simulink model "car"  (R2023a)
settings: Solver=ode15s  StartTime=0.0  StopTime=60  RelTol=1e-3  EnableMultiTasking=on
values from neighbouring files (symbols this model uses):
  A_a = 1.5    [modelparam.m]
  b_f = 0.1    [modelparam.m]
  b_t = 0.1    [modelparam.m]
  brake_gain = 1.0e3    (= 1000)    [modelparam.m]
  Bx = Kxk/(Cx*Dx)    (= 12.5)    [modelparam.m]
  c_c = 30    [modelparam.m]
  c_d = 1    [modelparam.m]
  c_p = 15    [modelparam.m]
  c_r = 0.015    [modelparam.m]
  c_w = 0.30    (= 0.3)    [modelparam.m]
  Cx = 1.2    [modelparam.m]
  Dx = muX*Fz    (= 5886)    [modelparam.m]
  Ex = 0.8    [modelparam.m]
  g = 9.81    [modelparam.m]
  gearInertia = [0.13 0.09 0.07 0.05 0.04]    [modelparam.m]
  gearNumber = [1 2 3 4 5]    [modelparam.m]
  gearRatio = [3.4 2.2 1.5 1.1 0.9]    [modelparam.m]
  i_f = 3.4    [modelparam.m]
  IdleControllerI = 0.2    [modelparam.m]
  IdleControllerP = 0.8    [modelparam.m]
  init_d = init_v/r_w/3.6    (= 27.7777777778)    [modelparam.m]
  init_e = init_t*gearRatio(2)    [modelparam.m]
  init_f = init_d    (= 27.7777777778)    [modelparam.m]
  init_t = init_f*i_f    (= 94.4444444444)    [modelparam.m]
  init_T = 0    [modelparam.m]
  J_e = 0.2    [modelparam.m]
  J_f = 0.1    [modelparam.m]
  J_w = 0.6    [modelparam.m]
  k_c = 10e3    (= 10000)    [modelparam.m]
  k_d = 1e3    (= 1000)    [modelparam.m]
  k_p = 0.5e4    (= 5000)    [modelparam.m]
  mass = 1.5e3    (= 1500)    [modelparam.m]
  N_idle = 8.5e2*pi/30    (= 89.0117918517)    [modelparam.m]
  N_max = 7e3*pi/30    (= 733.038285838)    [modelparam.m]
  position = [0 1e6]    [modelparam.m]
  r_w = 0.30    (= 0.3)    [modelparam.m]
  Rho_a = 1.29    [modelparam.m]
  slope = [0 0]    [modelparam.m]
  T_max = 400    [modelparam.m]
  tau_d = 1e-3    (= 0.001)    [modelparam.m]
  tau_e = 0.1    [modelparam.m]
libraries: simulink x4

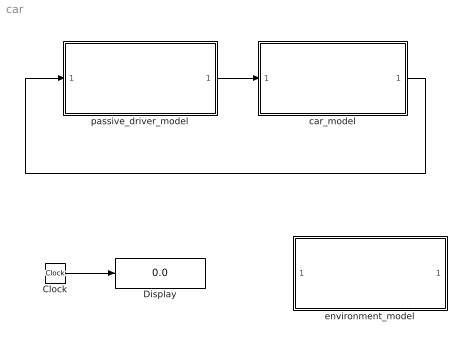
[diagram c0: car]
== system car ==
  Clock : Clock
  Display : Display
  car_model : Subsystem
  environment_model : Subsystem  AncestorBlock=capsim_lib/Environment/environment_model_jofr1  mask{Tamb=0, Pamb=0, pos=position, slope=slope}
      mask prompts: Tamb "Ambient Temperature [K]"; Pamb "Ambient Pressure [Pa]"; pos "positionvector in slope map [m]"; slope "slopevector in slope map [rad]"
      mask help: Environment settings
  passive_driver_model : Subsystem  AncestorBlock=capsim_lib/Driver/driver_model_template
      mask help: Driver model
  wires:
  car_model/1(vehicle fb out) -> passive_driver_model/1(vehicle fb in)
  passive_driver_model/1(driver cmd out) -> car_model/1(driver cmd in)
  Clock/1 -> Display/1

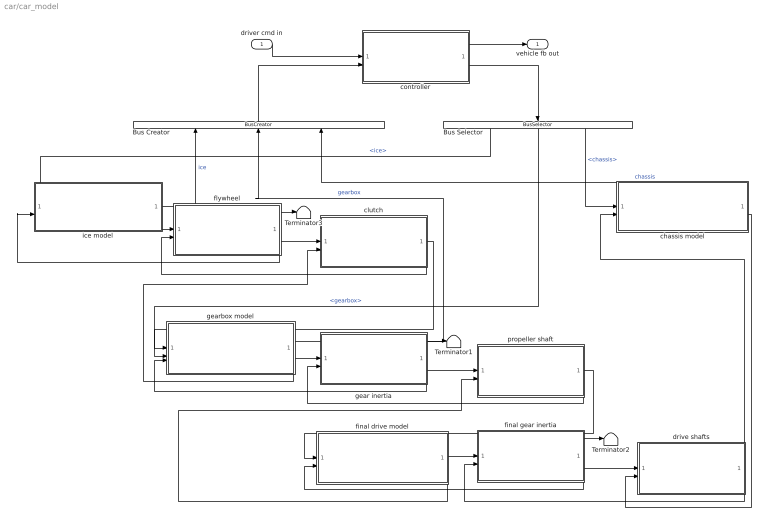
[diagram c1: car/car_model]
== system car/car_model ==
  driver cmd in : Inport
  Bus Creator : BusCreator  Inputs=3
  Bus Selector : BusSelector  OutputSignals=ice,gearbox,chassis
  Terminator1 : Terminator
  Terminator2 : Terminator
  Terminator3 : Terminator
  chassis model : Subsystem  AncestorBlock=capsim_lib/Chassis/chassis_model_template
  clutch : Subsystem  AncestorBlock=capsim_lib/MechConverter/mechconverter_simple1_std  mask{mass=0, inertia=0, k_c=k_c, c_c=c_c}
      mask prompts: mass "Component mass [kg]"; inertia "Inertia [kg*m2]"; k_c "stiffness [Nm/rad]"; c_c "damping [Nms/rad]"
      mask help: Inertia
  controller : Subsystem  AncestorBlock=capsim_lib/Controller/controller_template
  drive shafts : Subsystem  AncestorBlock=capsim_lib/MechConverter/mechconverter_simple1_std  mask{mass=0, inertia=0, k_d=k_d, c_d=c_d}
      mask prompts: mass "Component mass [kg]"; inertia "Inertia [kg*m2]"; k_d "stiffness [Nm/rad]"; c_d "damping [Nms/rad]"
      mask help: Inertia
  final drive model : Subsystem  AncestorBlock=capsim_lib/Gearbox/gearbox_template
  final gear inertia : Subsystem  AncestorBlock=capsim_lib/Inertia/inertia_simple1_std  mask{mass=0, inertia=0, speedinit=init_f, angleinit=0}
      mask prompts: mass "Component mass [kg]"; inertia "Inertia [kg*m2]"; speedinit "Initial speed [rad/s]"; angleinit "Initial angle [rad]"
      mask help: Inertia
  flywheel : Subsystem  AncestorBlock=capsim_lib/Inertia/inertia_simple1_std  mask{mass=0, inertia=0, speedinit=init_e, angleinit=0}
      mask prompts: mass "Component mass [kg]"; inertia "Inertia [kg*m2]"; speedinit "Initial speed [rad/s]"; angleinit "Initial angle [rad]"
      mask help: Inertia
  gear inertia : Subsystem  AncestorBlock=capsim_lib/Inertia/inertia_simple1_std  mask{mass=0, inertia=0, speedinit=init_t, angleinit=0}
      mask prompts: mass "Component mass [kg]"; inertia "Inertia [kg*m2]"; speedinit "Initial speed [rad/s]"; angleinit "Initial angle [rad]"
      mask help: Inertia
  gearbox model : Subsystem  AncestorBlock=capsim_lib/Gearbox/gearbox_template
  ice model : Subsystem
  propeller shaft : Subsystem  AncestorBlock=capsim_lib/MechConverter/mechconverter_simple1_std  mask{mass=0, inertia=0, k_p=k_p, c_p=c_p}
      mask prompts: mass "Component mass [kg]"; inertia "Inertia [kg*m2]"; k_p "stiffness [Nm/rad]"; c_p "damping [Nms/rad]"
      mask help: Inertia
  vehicle fb out : Outport
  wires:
  controller/1(vehicle fb out) -> vehicle fb out/1
  driver cmd in/1 -> controller/1(driver cmd in)
  controller/2(cmd out) -> Bus Selector/1
  Bus Creator/1 -> controller/2(sensor in)
  Bus Selector/1 -> ice model/1(cmd in)  "<ice>"
  Bus Selector/3 -> chassis model/1(cmd in)  "<chassis>"
  chassis model/1(sensor out) -> Bus Creator/3  "chassis"
  ice model/2(mech power out [Nm]) -> flywheel/1(mech in [Nm])
  flywheel/3(mech fb out [rad/s]) -> ice model/2(mech fb in [rad/s])
  flywheel/2(mech out [rad/s]) -> clutch/1(mech in [rad/s])
  clutch/2(mech fb out [Nm]) -> flywheel/2(mech fb in [Nm])
  clutch/1(mech out [Nm]) -> gearbox model/2(mech power in [Nm])
  gearbox model/2(mech power out [Nm]) -> gear inertia/1(mech in [Nm])
  gearbox model/3(mech fb out [rad/s]) -> clutch/2(mech fb in [rad/s])
  gear inertia/3(mech fb out [rad/s]) -> gearbox model/3(mech fb in [rad/s])
  gear inertia/2(mech out [rad/s]) -> propeller shaft/1(mech in [rad/s])
  propeller shaft/2(mech fb out [Nm]) -> gear inertia/2(mech fb in [Nm])
  propeller shaft/1(mech out [Nm]) -> final drive model/1(mech power in [Nm])
  final drive model/2(mech fb out [rad/s]) -> propeller shaft/2(mech fb in [rad/s])
  final drive model/1(mech power out [Nm]) -> final gear inertia/1(mech in [Nm])
  final gear inertia/2(mech out [rad/s]) -> drive shafts/1(mech in [rad/s])
  final gear inertia/3(mech fb out [rad/s]) -> final drive model/2(mech fb in [rad/s])
  drive shafts/1(mech out [Nm]) -> chassis model/2(mech power in [Nm])
  drive shafts/2(mech fb out [Nm]) -> final gear inertia/2(mech fb in [Nm])
  chassis model/2(mech fb out [rad/s]) -> drive shafts/2(mech fb in [rad/s])
  ice model/1(sensor out) -> Bus Creator/1  "ice"
  flywheel/1(sensor out) -> Terminator3/1
  gearbox model/1(sensor out) -> Bus Creator/2  "gearbox"
  gear inertia/1(sensor out) -> Terminator1/1
  final gear inertia/1(sensor out) -> Terminator2/1
  Bus Selector/2 -> gearbox model/1(cmd in)  "<gearbox>"

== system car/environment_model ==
  Compare To Constant : simulink/Logic and Bit Operations/Compare To Constant  relop=<  const=1  OutDataTypeStr=uint8  ZeroCross=off
  Compare To Constant1 : simulink/Logic and Bit Operations/Compare To Constant  relop=<  const=1  OutDataTypeStr=uint8  ZeroCross=off
  Constant2 : Constant  Value=pos(end)
  Integrator : Integrator
  Logical Operator : Logic  Operator=OR  Inputs=3  AllPortsSameDT=off  OutDataTypeStr=boolean
  Relational Operator : RelationalOperator
  Stop Simulation1 : Stop
  To Workspace2 : ToWorkspace  VariableName=environmentout  SampleTime=-1
  slope as function of the distance : Lookup  InputValues=pos  Table=slope  LookUpMeth=Interpolation-Use End Values
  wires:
  [speed] -> Integrator/1, Compare To Constant/1
  Integrator/1 -> slope as function of the distance/1, Relational Operator/1  "distance"
  slope as function of the distance/1 -> [slope], To Workspace2/1
  Constant2/1 -> Relational Operator/2
  Logical Operator/1 -> Stop Simulation1/1
  Relational Operator/1 -> Logical Operator/1
  Compare To Constant/1 -> Logical Operator/2
  [wheelspeed] -> Compare To Constant1/1
  Compare To Constant1/1 -> Logical Operator/3

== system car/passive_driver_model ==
  vehicle fb in : Inport
  Bus Creator : BusCreator  Inputs=1
  Bus Selector : BusSelector  OutputSignals=velocity [m/s]
  From Workspace2 : FromWorkspace  VariableName=[InputT InputU]
  Terminator : Terminator
  driver cmd out : Outport
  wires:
  vehicle fb in/1 -> Bus Selector/1
  Bus Creator/1 -> driver cmd out/1
  Bus Selector/1 -> Terminator/1  "<velocity [m/s]>"
  From Workspace2/1 -> Bus Creator/1  "Torque demand [%]"

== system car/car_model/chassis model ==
  cmd in : Inport
  mech power in [Nm] : Inport  Port=2
  chassis : Subsystem  mask{g=g, mass=mass, J_w=J_w, r_w=r_w, init_d=init_d, c_w=c_w, A_a=A_a, Rho_a=Rho_a, c_r=c_r, Bx=Bx, Cx=Cx, Dx=Dx, Ex=Ex}
      mask prompts: g "gravity constant [m/s^2]"; mass "vehicle mass [kg]"; J_w "wheel inertia [kg m^2]"; r_w "wheel radius [m]"; init_d "initial drive shaft speed [rad/s]"; c_w "air drag coefficient [-]"; A_a "max. vehicle cross section area [m^2]"; Rho_a "Air density [kg/m^3]"; c_r "rolling resistance coefficient [-]"; Bx "Magic Bx"; Cx "Magic Cx"; Dx "Magic Dx"; Ex "Magic Ex"
  local controller : Subsystem  mask{brake_gain=brake_gain}
      mask prompts: brake_gain "brake gain [Nm]"
  sensor out : Outport
  mech fb out [rad/s] : Outport  Port=2
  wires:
  local controller/2(ctrl out) -> chassis/1(ctrl in)
  cmd in/1 -> local controller/1(cmd in)
  local controller/1(sensor out) -> sensor out/1
  chassis/1(sensor out) -> local controller/2(sensor in)
  mech power in [Nm]/1 -> chassis/2(mech power in [Nm])
  chassis/2(mech fb out [rad/s]) -> mech fb out [rad/s]/1

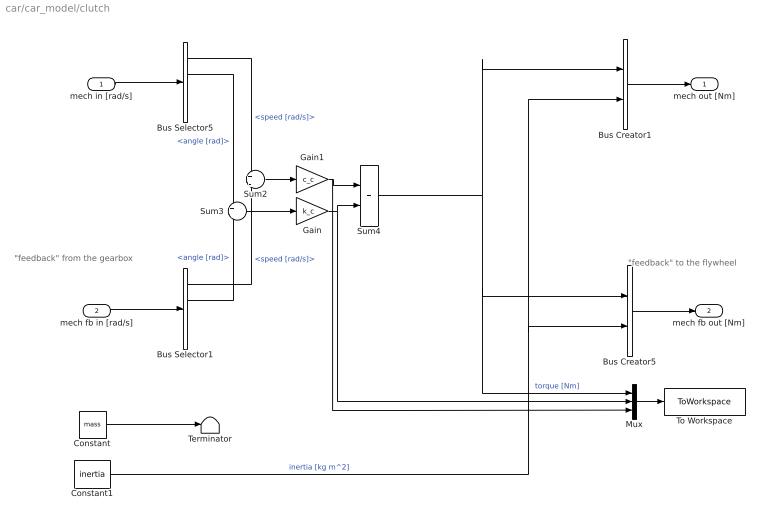
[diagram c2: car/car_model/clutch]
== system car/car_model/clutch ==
  note: "feedback" from the gearbox
  note: "feedback" to the flywheel
  mech in [rad/s] : Inport
  mech fb in [rad/s] : Inport  Port=2
  Bus Creator1 : BusCreator  Inputs=2
  Bus Creator5 : BusCreator  Inputs=2
  Bus Selector1 : BusSelector  OutputSignals=speed [rad/s],angle [rad]
  Bus Selector5 : BusSelector  OutputSignals=speed [rad/s],angle [rad]
  Constant : Constant  Value=mass
  Constant1 : Constant  Value=inertia
  Gain : Gain  Gain=k_c
  Gain1 : Gain  Gain=c_c
  Mux : Mux  Inputs=3
  Sum2 : Sum  Inputs=+|-  SaturateOnIntegerOverflow=on
  Sum3 : Sum  Inputs=+|-  SaturateOnIntegerOverflow=on
  Sum4 : Sum
  Terminator : Terminator
  To Workspace : ToWorkspace  VariableName=clutchout  SampleTime=-1
  mech out [Nm] : Outport
  mech fb out [Nm] : Outport  Port=2
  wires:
  mech in [rad/s]/1 -> Bus Selector5/1
  mech fb in [rad/s]/1 -> Bus Selector1/1
  Mux/1 -> To Workspace/1
  Constant/1 -> Terminator/1
  Bus Creator5/1 -> mech fb out [Nm]/1
  Bus Creator1/1 -> mech out [Nm]/1
  Bus Selector5/1 -> Sum2/1  "<speed [rad/s]>"
  Bus Selector5/2 -> Sum3/1  "<angle [rad]>"
  Bus Selector1/1 -> Sum2/2  "<speed [rad/s]>"
  Bus Selector1/2 -> Sum3/2  "<angle [rad]>"
  Sum2/1 -> Gain1/1
  Sum3/1 -> Gain/1
  Gain1/1 -> Sum4/1, Mux/3
  Gain/1 -> Sum4/2, Mux/2
  Sum4/1 -> Bus Creator1/1, Bus Creator5/1, Mux/1  "torque [Nm]"
  Constant1/1 -> Bus Creator5/2, Bus Creator1/2  "inertia [kg m^2]"

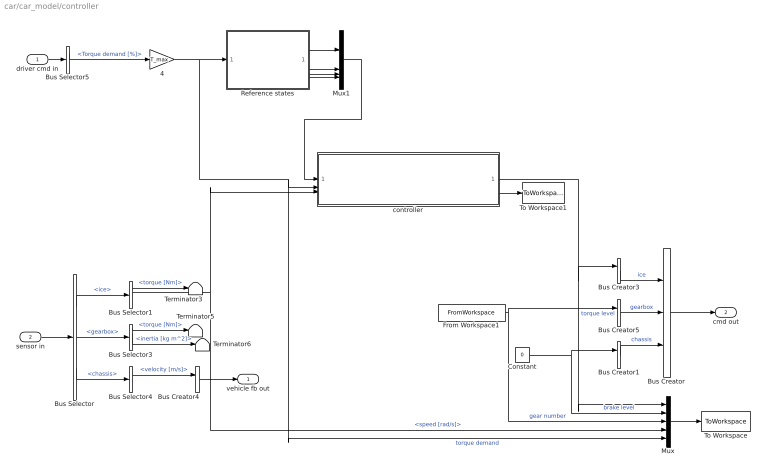
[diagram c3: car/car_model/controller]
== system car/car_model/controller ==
  driver cmd in : Inport
  sensor in : Inport  Port=2
  4 : Gain  Gain=T_max
  Bus Creator : BusCreator  Inputs=3
  Bus Creator{1,3..5} (4 alike) : BusCreator  Inputs=1
  Bus Selector : BusSelector  OutputSignals=ice,gearbox,chassis
  Bus Selector1 : BusSelector  OutputSignals=torque [Nm],speed [rad/s]
  Bus Selector3 : BusSelector  OutputSignals=torque [Nm],inertia [kg m^2]
  Bus Selector4 : BusSelector  OutputSignals=velocity [m/s]
  Bus Selector5 : BusSelector  OutputSignals=Torque demand [%]
  Constant : Constant  Value=0
  From Workspace1 : FromWorkspace  VariableName=[InputT InputG]
  Mux : Mux  Inputs=5
  Mux1 : Mux
  Reference states : Subsystem
  Terminator3 : Terminator
  Terminator5 : Terminator
  Terminator6 : Terminator
  To Workspace : ToWorkspace  VariableName=controllerout  SampleTime=-1
  To Workspace1 : ToWorkspace  VariableName=obsstates  SampleTime=-1
  controller : Subsystem
  vehicle fb out : Outport
  cmd out : Outport  Port=2
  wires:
  Bus Creator/1 -> cmd out/1
  Bus Creator3/1 -> Bus Creator/1  "ice"
  sensor in/1 -> Bus Selector/1
  Bus Selector/1 -> Bus Selector1/1  "<ice>"
  driver cmd in/1 -> Bus Selector5/1
  Bus Creator4/1 -> vehicle fb out/1
  Bus Selector5/1 -> 4/1  "<Torque demand [%]>"
  Bus Selector3/1 -> Terminator5/1  "<torque [Nm]>"
  Bus Selector3/2 -> Terminator6/1  "<inertia [kg m^2]>"
  Mux/1 -> To Workspace/1
  Bus Creator1/1 -> Bus Creator/3  "chassis"
  Bus Selector/2 -> Bus Selector3/1  "<gearbox>"
  Bus Selector/3 -> Bus Selector4/1  "<chassis>"
  Bus Selector1/1 -> Terminator3/1  "<torque [Nm]>"
  Bus Selector1/2 -> Mux/4, controller/3(Engine speed sensor)  "<speed [rad/s]>"
  Bus Selector4/1 -> Bus Creator4/1  "<velocity [m/s]>"
  Constant/1 -> Bus Creator1/1, Mux/2  "brake level"
  From Workspace1/1 -> Bus Creator5/1, Mux/3  "gear number"
  Bus Creator5/1 -> Bus Creator/2  "gearbox"
  4/1 -> Reference states/1(In1), Mux/5, controller/2(Torque demand from driver)  "torque demand"
  Reference states/1(Drive shaft torsion [rad]) -> Mux1/1
  Reference states/2(Engine speed [rad/s]) -> Mux1/2
  Reference states/3(Wheel speed [rad/s]) -> Mux1/3
  Reference states/4(Engine torque [Nm]) -> Mux1/4
  Mux1/1 -> controller/1(x_ref)
  controller/1(Torque demand from controller) -> Mux/1, Bus Creator3/1  "torque level"
  controller/2(Observed states) -> To Workspace1/1

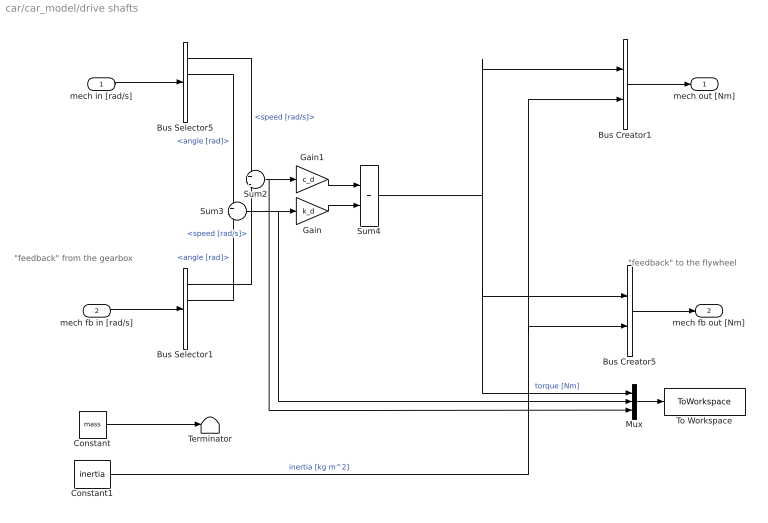
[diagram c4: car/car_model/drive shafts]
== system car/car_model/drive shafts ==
  note: "feedback" from the gearbox
  note: "feedback" to the flywheel
  mech in [rad/s] : Inport
  mech fb in [rad/s] : Inport  Port=2
  Bus Creator1 : BusCreator  Inputs=2
  Bus Creator5 : BusCreator  Inputs=2
  Bus Selector1 : BusSelector  OutputSignals=speed [rad/s],angle [rad]
  Bus Selector5 : BusSelector  OutputSignals=speed [rad/s],angle [rad]
  Constant : Constant  Value=mass
  Constant1 : Constant  Value=inertia
  Gain : Gain  Gain=k_d
  Gain1 : Gain  Gain=c_d
  Mux : Mux  Inputs=3
  Sum2 : Sum  Inputs=+|-  SaturateOnIntegerOverflow=on
  Sum3 : Sum  Inputs=+|-  SaturateOnIntegerOverflow=on
  Sum4 : Sum
  Terminator : Terminator
  To Workspace : ToWorkspace  VariableName=driveshaftsout  SampleTime=-1
  mech out [Nm] : Outport
  mech fb out [Nm] : Outport  Port=2
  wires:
  mech in [rad/s]/1 -> Bus Selector5/1
  mech fb in [rad/s]/1 -> Bus Selector1/1
  Mux/1 -> To Workspace/1
  Constant/1 -> Terminator/1
  Bus Creator5/1 -> mech fb out [Nm]/1
  Bus Creator1/1 -> mech out [Nm]/1
  Bus Selector5/1 -> Sum2/1  "<speed [rad/s]>"
  Bus Selector5/2 -> Sum3/1  "<angle [rad]>"
  Bus Selector1/1 -> Sum2/2  "<speed [rad/s]>"
  Bus Selector1/2 -> Sum3/2  "<angle [rad]>"
  Sum2/1 -> Gain1/1, Mux/3
  Sum3/1 -> Gain/1, Mux/2
  Gain1/1 -> Sum4/1
  Gain/1 -> Sum4/2
  Sum4/1 -> Bus Creator1/1, Bus Creator5/1, Mux/1  "torque [Nm]"
  Constant1/1 -> Bus Creator5/2, Bus Creator1/2  "inertia [kg m^2]"

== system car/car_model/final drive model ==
  mech power in [Nm] : Inport
  mech fb in [rad/s] : Inport  Port=2
  final_drive : Subsystem  mask{mass=0, inertia=J_f, b_f=b_f, i_f=i_f}
      mask prompts: mass "mass [kg]"; inertia "inertia [kg m^2]"; b_f "Damping [Nm s/rad]"; i_f "Ratio [-]"
  mech power out [Nm] : Outport
  mech fb out [rad/s] : Outport  Port=2
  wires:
  mech fb in [rad/s]/1 -> final_drive/2(mech fb in [rad/s])
  final_drive/1(mech power out [Nm]) -> mech power out [Nm]/1
  mech power in [Nm]/1 -> final_drive/1(mech power in [Nm])
  final_drive/2(mech fb out [rad/s]) -> mech fb out [rad/s]/1

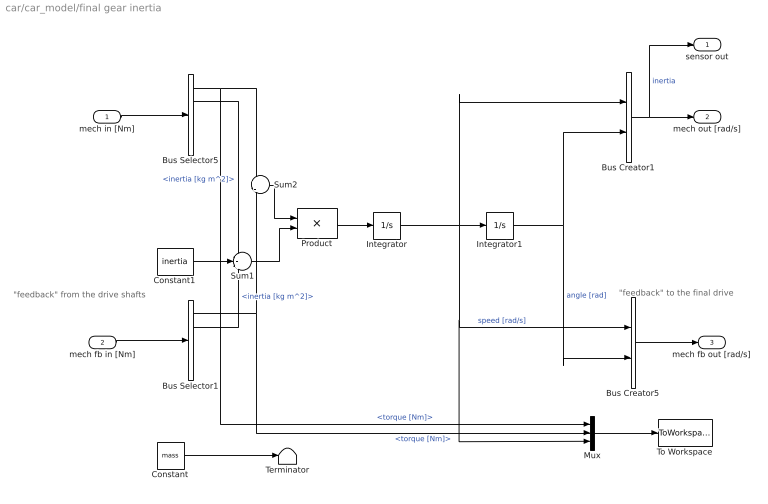
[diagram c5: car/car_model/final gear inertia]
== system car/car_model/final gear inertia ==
  note: "feedback" to the final drive
  note: "feedback" from the drive shafts
  mech in [Nm] : Inport
  mech fb in [Nm] : Inport  Port=2
  Bus Creator1 : BusCreator  Inputs=2
  Bus Creator5 : BusCreator  Inputs=2
  Bus Selector1 : BusSelector  OutputSignals=torque [Nm],inertia [kg m^2]
  Bus Selector5 : BusSelector  OutputSignals=torque [Nm],inertia [kg m^2]
  Constant : Constant  Value=mass
  Constant1 : Constant  Value=inertia
  Integrator : Integrator  InitialCondition=speedinit
  Integrator1 : Integrator  InitialCondition=angleinit
  Mux : Mux  Inputs=3
  Product : Product  Inputs=*/  SaturateOnIntegerOverflow=on
  Sum1 : Sum  Inputs=+++  SaturateOnIntegerOverflow=on
  Sum2 : Sum  Inputs=+|-  SaturateOnIntegerOverflow=on
  Terminator : Terminator
  To Workspace : ToWorkspace  VariableName=finalgearout  SampleTime=-1
  sensor out : Outport
  mech out [rad/s] : Outport  Port=2
  mech fb out [rad/s] : Outport  Port=3
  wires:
  Constant1/1 -> Sum1/2
  Bus Selector1/2 -> Sum1/3  "<inertia [kg m^2]>"
  Bus Selector1/1 -> Sum2/2, Mux/2  "<torque [Nm]>"
  Bus Selector5/2 -> Sum1/1  "<inertia [kg m^2]>"
  Bus Selector5/1 -> Sum2/1, Mux/1  "<torque [Nm]>"
  Bus Creator1/1 -> sensor out/1, mech out [rad/s]/1  "inertia"
  Bus Creator5/1 -> mech fb out [rad/s]/1
  mech fb in [Nm]/1 -> Bus Selector1/1
  Constant/1 -> Terminator/1
  mech in [Nm]/1 -> Bus Selector5/1
  Integrator1/1 -> Bus Creator5/2, Bus Creator1/2  "angle [rad]"
  Integrator/1 -> Bus Creator1/1, Integrator1/1, Bus Creator5/1, Mux/3  "speed [rad/s]"
  Product/1 -> Integrator/1
  Sum1/1 -> Product/2
  Sum2/1 -> Product/1
  Mux/1 -> To Workspace/1

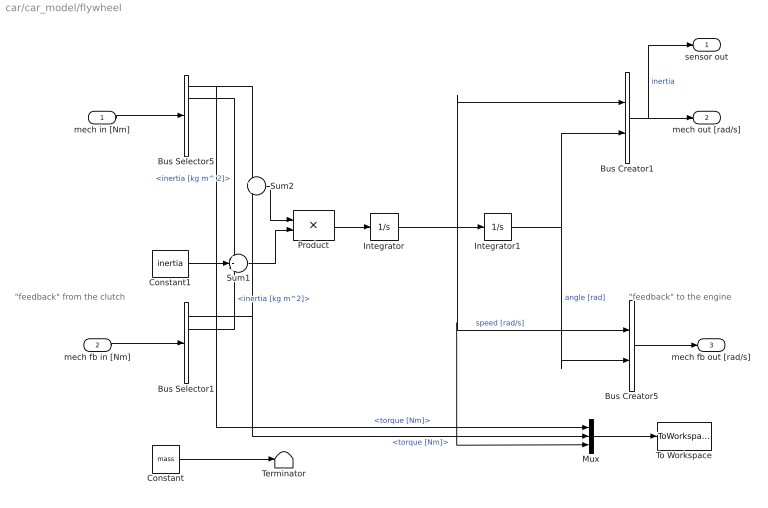
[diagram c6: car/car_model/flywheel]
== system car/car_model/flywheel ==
  note: "feedback" to the engine
  note: "feedback" from the clutch
  mech in [Nm] : Inport
  mech fb in [Nm] : Inport  Port=2
  Bus Creator1 : BusCreator  Inputs=2
  Bus Creator5 : BusCreator  Inputs=2
  Bus Selector1 : BusSelector  OutputSignals=torque [Nm],inertia [kg m^2]
  Bus Selector5 : BusSelector  OutputSignals=torque [Nm],inertia [kg m^ 2]
  Constant : Constant  Value=mass
  Constant1 : Constant  Value=inertia
  Integrator : Integrator  InitialCondition=speedinit
  Integrator1 : Integrator  InitialCondition=angleinit
  Mux : Mux  Inputs=3
  Product : Product  Inputs=*/  SaturateOnIntegerOverflow=on
  Sum1 : Sum  Inputs=+++  SaturateOnIntegerOverflow=on
  Sum2 : Sum  Inputs=+|-  SaturateOnIntegerOverflow=on
  Terminator : Terminator
  To Workspace : ToWorkspace  VariableName=flywheelout  SampleTime=-1
  sensor out : Outport
  mech out [rad/s] : Outport  Port=2
  mech fb out [rad/s] : Outport  Port=3
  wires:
  Mux/1 -> To Workspace/1
  Sum2/1 -> Product/1
  Sum1/1 -> Product/2
  Product/1 -> Integrator/1
  Integrator/1 -> Mux/3, Bus Creator5/1, Integrator1/1, Bus Creator1/1  "speed [rad/s]"
  Integrator1/1 -> Bus Creator5/2, Bus Creator1/2  "angle [rad]"
  mech in [Nm]/1 -> Bus Selector5/1
  Constant/1 -> Terminator/1
  mech fb in [Nm]/1 -> Bus Selector1/1
  Bus Creator5/1 -> mech fb out [rad/s]/1
  Bus Creator1/1 -> mech out [rad/s]/1, sensor out/1  "inertia"
  Bus Selector5/1 -> Mux/1, Sum2/1  "<torque [Nm]>"
  Bus Selector5/2 -> Sum1/1  "<inertia [kg m^ 2]>"
  Bus Selector1/1 -> Mux/2, Sum2/2  "<torque [Nm]>"
  Bus Selector1/2 -> Sum1/3  "<inertia [kg m^2]>"
  Constant1/1 -> Sum1/2

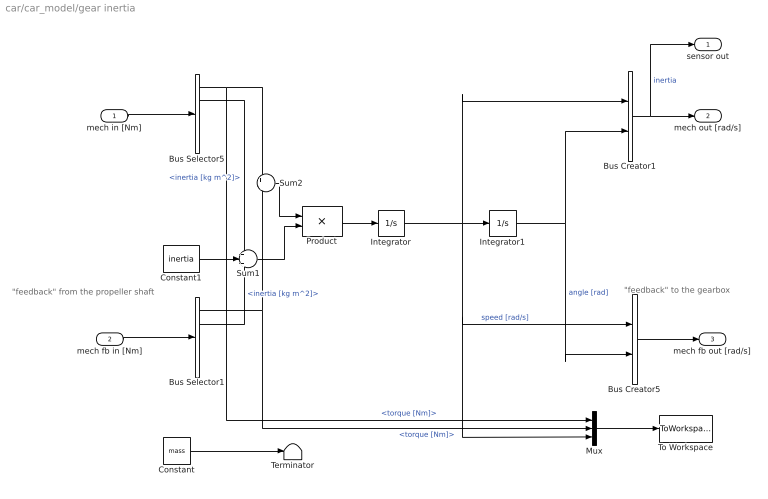
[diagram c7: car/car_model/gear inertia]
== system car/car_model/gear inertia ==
  note: "feedback" from the propeller shaft
  note: "feedback" to the gearbox
  mech in [Nm] : Inport
  mech fb in [Nm] : Inport  Port=2
  Bus Creator1 : BusCreator  Inputs=2
  Bus Creator5 : BusCreator  Inputs=2
  Bus Selector1 : BusSelector  OutputSignals=torque [Nm],inertia [kg m^2]
  Bus Selector5 : BusSelector  OutputSignals=torque [Nm],inertia [kg m^2]
  Constant : Constant  Value=mass
  Constant1 : Constant  Value=inertia
  Integrator : Integrator  InitialCondition=speedinit
  Integrator1 : Integrator  InitialCondition=angleinit
  Mux : Mux  Inputs=3
  Product : Product  Inputs=*/  SaturateOnIntegerOverflow=on
  Sum1 : Sum  Inputs=+++  SaturateOnIntegerOverflow=on
  Sum2 : Sum  Inputs=+|-  SaturateOnIntegerOverflow=on
  Terminator : Terminator
  To Workspace : ToWorkspace  VariableName=gearinertiaout  SampleTime=-1
  sensor out : Outport
  mech out [rad/s] : Outport  Port=2
  mech fb out [rad/s] : Outport  Port=3
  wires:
  Mux/1 -> To Workspace/1
  Sum2/1 -> Product/1
  Sum1/1 -> Product/2
  Product/1 -> Integrator/1
  Integrator/1 -> Mux/3, Bus Creator5/1, Integrator1/1, Bus Creator1/1  "speed [rad/s]"
  Integrator1/1 -> Bus Creator5/2, Bus Creator1/2  "angle [rad]"
  mech in [Nm]/1 -> Bus Selector5/1
  Constant/1 -> Terminator/1
  mech fb in [Nm]/1 -> Bus Selector1/1
  Bus Creator5/1 -> mech fb out [rad/s]/1
  Bus Creator1/1 -> mech out [rad/s]/1, sensor out/1  "inertia"
  Bus Selector5/1 -> Mux/1, Sum2/1  "<torque [Nm]>"
  Bus Selector5/2 -> Sum1/1  "<inertia [kg m^2]>"
  Bus Selector1/1 -> Mux/2, Sum2/2  "<torque [Nm]>"
  Bus Selector1/2 -> Sum1/3  "<inertia [kg m^2]>"
  Constant1/1 -> Sum1/2

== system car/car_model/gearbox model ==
  cmd in : Inport
  mech power in [Nm] : Inport  Port=2
  mech fb in [rad/s] : Inport  Port=3
  gearbox : Subsystem  mask{mass=0, inertia=0, b_t=b_t}
      mask prompts: mass "mass [kg]"; inertia "inertia [kg m^2]"; b_t "Damping [Nm s/rad]"
  local controller : Subsystem  mask{gearNumber=gearNumber, gearRatio=gearRatio, gearInertia=gearInertia}
      mask prompts: gearNumber "gear number vector"; gearRatio "gear ratio vector"; gearInertia "gear inertia vector"
  sensor out : Outport
  mech power out [Nm] : Outport  Port=2
  mech fb out [rad/s] : Outport  Port=3
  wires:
  gearbox/3(mech fb out [rad/s]) -> mech fb out [rad/s]/1
  mech power in [Nm]/1 -> gearbox/2(mech power in [Nm])
  gearbox/2(mech power out [Nm]) -> mech power out [Nm]/1
  mech fb in [rad/s]/1 -> gearbox/3(mech fb in [rad/s])
  gearbox/1(sensor out) -> local controller/2(sensor in)
  local controller/1(sensor out) -> sensor out/1
  cmd in/1 -> local controller/1(cmd in)
  local controller/2(ctrl) -> gearbox/1(ctrl)

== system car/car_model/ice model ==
  cmd in : Inport
  mech fb in [rad/s] : Inport  Port=2
  ice : Subsystem  mask{mass=0, inertia=J_e, tau_d=tau_d, tau_e=tau_e, init_T=init_T}
      mask prompts: mass "mass [kg]"; inertia "inertia [kg m^2]"; tau_d "time delay [s]"; tau_e "time constant [s]"; init_T "initial torque [Nm]"
  local controller : Subsystem  mask{T_max=T_max, N_max=N_max, N_idle=N_idle, P=IdleControllerP, I=IdleControllerI}
      mask prompts: T_max "maximum torque [Nm]"; N_max "maximum speed [rad/s]"; N_idle "Idle controller reference value [rad/s]"; P "Idle controller proportional gain"; I "Idle controller integral gain"
  sensor out : Outport
  mech power out [Nm] : Outport  Port=2
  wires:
  ice/2(mech power out [Nm]) -> mech power out [Nm]/1
  mech fb in [rad/s]/1 -> ice/2(mech fb in [rad/s])
  ice/1(sensor out) -> local controller/2(sensor in)
  local controller/1(sensor out) -> sensor out/1
  cmd in/1 -> local controller/1(cmd in)
  local controller/2(ctrl) -> ice/1(ctrl)

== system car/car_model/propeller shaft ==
  note: "feedback" to the flywheel
  note: "feedback" from the gearbox
  mech in [rad/s] : Inport
  mech fb in [rad/s] : Inport  Port=2
  Bus Creator1 : BusCreator  Inputs=2
  Bus Creator5 : BusCreator  Inputs=2
  Bus Selector1 : BusSelector  OutputSignals=speed [rad/s],angle [rad]
  Bus Selector5 : BusSelector  OutputSignals=speed [rad/s],angle [rad]
  Constant : Constant  Value=mass
  Constant1 : Constant  Value=inertia
  Gain : Gain  Gain=k_p
  Gain1 : Gain  Gain=c_p
  Mux : Mux  Inputs=3
  Sum2 : Sum  Inputs=+|-  SaturateOnIntegerOverflow=on
  Sum3 : Sum  Inputs=+|-  SaturateOnIntegerOverflow=on
  Sum4 : Sum
  Terminator : Terminator
  To Workspace : ToWorkspace  VariableName=propellershaftout  SampleTime=-1
  mech out [Nm] : Outport
  mech fb out [Nm] : Outport  Port=2
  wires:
  Constant1/1 -> Bus Creator1/2, Bus Creator5/2  "inertia [kg m^2]"
  Sum4/1 -> Mux/1, Bus Creator5/1, Bus Creator1/1  "torque [Nm]"
  Gain/1 -> Sum4/2, Mux/2
  Gain1/1 -> Sum4/1, Mux/3
  Sum3/1 -> Gain/1
  Sum2/1 -> Gain1/1
  Bus Selector1/2 -> Sum3/2  "<angle [rad]>"
  Bus Selector1/1 -> Sum2/2  "<speed [rad/s]>"
  Bus Selector5/2 -> Sum3/1  "<angle [rad]>"
  Bus Selector5/1 -> Sum2/1  "<speed [rad/s]>"
  Bus Creator1/1 -> mech out [Nm]/1
  Bus Creator5/1 -> mech fb out [Nm]/1
  Constant/1 -> Terminator/1
  Mux/1 -> To Workspace/1
  mech fb in [rad/s]/1 -> Bus Selector1/1
  mech in [rad/s]/1 -> Bus Selector5/1

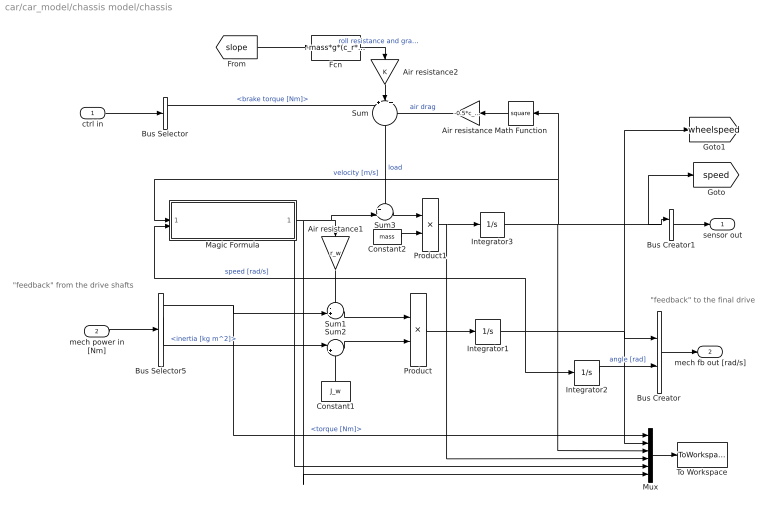
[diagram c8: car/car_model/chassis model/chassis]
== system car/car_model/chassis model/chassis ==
  note: "feedback" from the drive shafts
  note: "feedback" to the final drive
  ctrl in : Inport
  mech power in [Nm] : Inport  Port=2
  Air resistance : Gain  Gain=-0.5*c_w*A_a*Rho_a  SaturateOnIntegerOverflow=on
  Air resistance1 : Gain  Gain=r_w  SaturateOnIntegerOverflow=on
  Air resistance2 : Gain  SaturateOnIntegerOverflow=on
  Bus Creator : BusCreator  Inputs=2
  Bus Creator1 : BusCreator  Inputs=1
  Bus Selector : BusSelector  OutputSignals=brake torque [Nm]
  Bus Selector5 : BusSelector  OutputSignals=torque [Nm],inertia [kg m^2]
  Constant1 : Constant  Value=J_w
  Constant2 : Constant  Value=mass
  Fcn : Fcn  Expr=-mass*g*(c_r*cos(u) + sin(u))
  Integrator1 : Integrator  InitialCondition=init_d
  Integrator2 : Integrator
  Integrator3 : Integrator  InitialCondition=init_d*r_w
  Magic Formula : Subsystem
  Math Function : Math  Operator=square  SignedPower=on
  Mux : Mux  Inputs=6
  Product : Product  Inputs=*/  SaturateOnIntegerOverflow=on
  Product1 : Product  Inputs=*/  SaturateOnIntegerOverflow=on
  Sum : Sum  Inputs=+|+|+  SaturateOnIntegerOverflow=on
  Sum1 : Sum  Inputs=-+|  SaturateOnIntegerOverflow=on
  Sum2 : Sum  Inputs=|++  SaturateOnIntegerOverflow=on
  Sum3 : Sum  Inputs=++|  SaturateOnIntegerOverflow=on
  To Workspace : ToWorkspace  VariableName=chassisout  SampleTime=-1
  sensor out : Outport
  mech fb out [rad/s] : Outport  Port=2
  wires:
  Mux/1 -> To Workspace/1
  Integrator2/1 -> Bus Creator/2  "angle [rad]"
  Bus Selector5/2 -> Sum2/1  "<inertia [kg m^2]>"
  Bus Selector5/1 -> Mux/1, Sum1/2  "<torque [Nm]>"
  mech power in [Nm]/1 -> Bus Selector5/1
  Bus Creator/1 -> mech fb out [rad/s]/1
  ctrl in/1 -> Bus Selector/1
  [slope] -> Fcn/1
  Math Function/1 -> Air resistance/1
  Integrator1/1 -> Integrator2/1, Magic Formula/2(wheel speed [rad/s]), Mux/2, Bus Creator/1, [wheelspeed]  "speed [rad/s]"
  Air resistance/1 -> Sum/3  "air drag"
  Fcn/1 -> Air resistance2/1  "roll resistance and gravity"
  Bus Selector/1 -> Sum/1  "<brake torque [Nm]>"
  Bus Creator1/1 -> sensor out/1
  Sum2/1 -> Product/2
  Sum1/1 -> Product/1
  Product/1 -> Integrator1/1
  Constant1/1 -> Sum2/2
  Sum/1 -> Sum3/1  "load"
  Magic Formula/1(F_w [N]) -> Sum3/2, Air resistance1/1, Mux/6
  Sum3/1 -> Product1/1
  Constant2/1 -> Product1/2
  Product1/1 -> Integrator3/1, Mux/4
  Integrator3/1 -> Mux/3, Math Function/1, Magic Formula/1(forward velocity [m/s]), Bus Creator1/1, [speed]  "velocity [m/s]"
  Air resistance1/1 -> Sum1/1
  Magic Formula/2(slip ratio) -> Mux/5
  Air resistance2/1 -> Sum/2

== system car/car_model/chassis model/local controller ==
  cmd in : Inport
  sensor in : Inport  Port=2
  Bus Creator : BusCreator  Inputs=1
  Bus Selector : BusSelector  OutputSignals=brake level
  Saturation : Saturate  UpperLimit=1  LowerLimit=0
  brake_gain : Gain  Gain=-brake_gain  SaturateOnIntegerOverflow=on
  sensor out : Outport
  ctrl out : Outport  Port=2
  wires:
  cmd in/1 -> Bus Selector/1
  Bus Selector/1 -> Saturation/1  "<brake level>"
  Saturation/1 -> brake_gain/1
  brake_gain/1 -> Bus Creator/1  "brake torque [Nm]"
  Bus Creator/1 -> ctrl out/1
  sensor in/1 -> sensor out/1

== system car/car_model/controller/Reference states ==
  In1 : Inport
  1 : Gain  Gain=i_f*gearRatio(1)
  2 : Gain  Gain=1/tau_e
  5 : Gain  Gain=1/r_w
  6 : Gain  Gain=i_f*gearRatio(1)/k_d
  Add : Sum  Inputs=+-
  Fcn : Fcn  Expr=(i_f*gearRatio(1)/r_w*u(1)-0.5*Rho_a*c_w*A_a*u(2)^2-mass*g*c_r)/(mass+i_f^2*gearRatio(1)^2/r_w^2*J_e)
  Integrator : Integrator  InitialCondition=28/3.6
  Integrator1 : Integrator  InitialCondition=-8
  Mux6 : Mux  Inputs=2
  Drive shaft torsion [rad] : Outport
  Engine speed [rad/s] : Outport  Port=2
  Wheel speed [rad/s] : Outport  Port=3
  Engine torque [Nm] : Outport  Port=4
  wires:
  Fcn/1 -> Integrator/1
  Integrator/1 -> Mux6/2, 5/1  "v"
  Mux6/1 -> Fcn/1
  5/1 -> Wheel speed [rad/s]/1, 1/1
  6/1 -> Drive shaft torsion [rad]/1
  1/1 -> Engine speed [rad/s]/1
  Integrator1/1 -> Mux6/1, Engine torque [Nm]/1, 6/1, Add/2
  In1/1 -> Add/1
  Add/1 -> 2/1
  2/1 -> Integrator1/1

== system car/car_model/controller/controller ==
  note: Construct an observer for the vehicle using the engine speed sensor. Then use the given reference states (x_ref) and design a state feedback controller to damp the driveline oscillations.
  note: Connect your observed states here to plot them in Figure 3
  x_ref : Inport
  Torque demand from driver : Inport  Port=2
  Engine speed sensor : Inport  Port=3
  Ground : Ground
  Ground1 : Ground
  Manual Switch : ManualSwitch
  Mux : Mux
  Saturation : Saturate  UpperLimit=T_max  LowerLimit=-T_max
  Terminator1 : Terminator
  Terminator3 : Terminator
  Torque demand from controller : Outport
  Observed states : Outport  Port=2
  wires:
  Torque demand from driver/1 -> Manual Switch/1
  Manual Switch/1 -> Saturation/1
  Engine speed sensor/1 -> Terminator3/1
  x_ref/1 -> Terminator1/1
  Ground/1 -> Manual Switch/2
  Ground1/1 -> Mux/1, Mux/2, Mux/3, Mux/4
  Mux/1 -> Observed states/1
  Saturation/1 -> Torque demand from controller/1

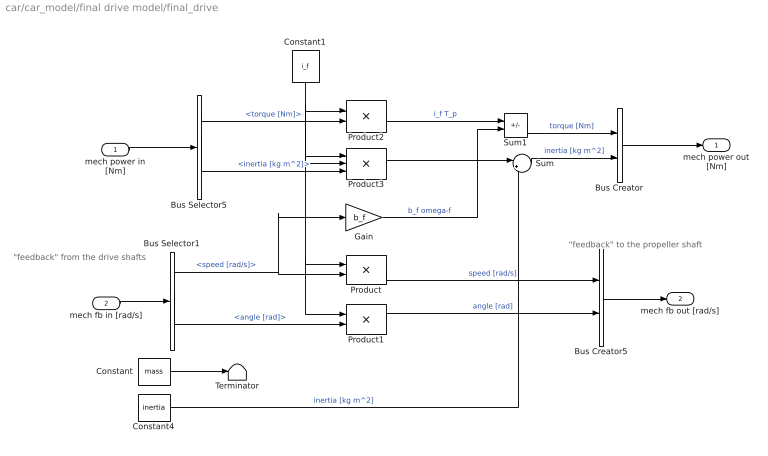
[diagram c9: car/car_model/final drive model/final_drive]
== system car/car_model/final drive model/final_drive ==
  note: "feedback" to the propeller shaft
  note: "feedback" from the drive shafts
  mech power in [Nm] : Inport
  mech fb in [rad/s] : Inport  Port=2
  Bus Creator : BusCreator  Inputs=2
  Bus Creator5 : BusCreator  Inputs=2
  Bus Selector1 : BusSelector  OutputSignals=speed [rad/s],angle [rad]
  Bus Selector5 : BusSelector  OutputSignals=torque [Nm],inertia [kg m^2]
  Constant : Constant  Value=mass
  Constant1 : Constant  Value=i_f
  Constant4 : Constant  Value=inertia
  Gain : Gain  Gain=b_f
  Product : Product  Inputs=**  SaturateOnIntegerOverflow=on
  Product1 : Product  Inputs=**  SaturateOnIntegerOverflow=on
  Product2 : Product  SaturateOnIntegerOverflow=on
  Product3 : Product  Inputs=3  SaturateOnIntegerOverflow=on
  Sum : Sum  Inputs=|++
  Sum1 : Sum  Inputs=+-
  Terminator : Terminator
  mech power out [Nm] : Outport
  mech fb out [rad/s] : Outport  Port=2
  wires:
  Gain/1 -> Sum1/2  "b_f omega-f"
  Sum1/1 -> Bus Creator/1  "torque [Nm]"
  Product2/1 -> Sum1/1  "i_f T_p"
  Sum/1 -> Bus Creator/2  "inertia [kg m^2]"
  Product3/1 -> Sum/1
  Constant4/1 -> Sum/2  "inertia [kg m^2]"
  Constant1/1 -> Product3/2, Product3/1, Product2/1, Product1/1, Product/1
  mech fb in [rad/s]/1 -> Bus Selector1/1
  Bus Creator/1 -> mech power out [Nm]/1
  Bus Selector1/2 -> Product1/2  "<angle [rad]>"
  Constant/1 -> Terminator/1
  Bus Selector1/1 -> Gain/1, Product/2  "<speed [rad/s]>"
  mech power in [Nm]/1 -> Bus Selector5/1
  Bus Selector5/1 -> Product2/2  "<torque [Nm]>"
  Bus Selector5/2 -> Product3/3  "<inertia [kg m^2]>"
  Product/1 -> Bus Creator5/1  "speed [rad/s]"
  Product1/1 -> Bus Creator5/2  "angle [rad]"
  Bus Creator5/1 -> mech fb out [rad/s]/1

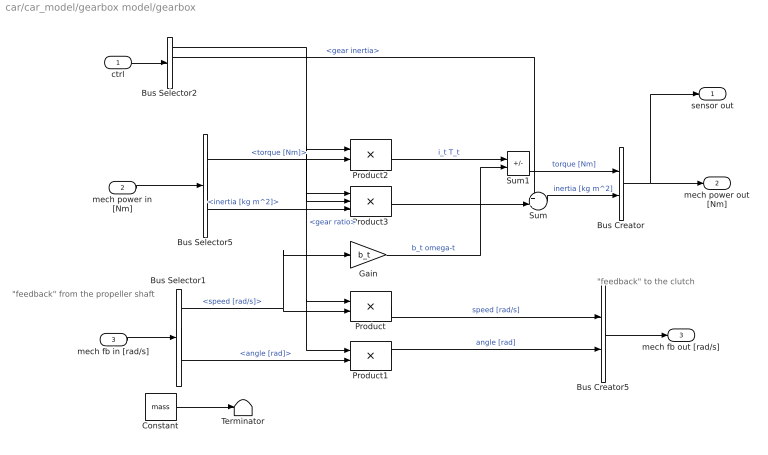
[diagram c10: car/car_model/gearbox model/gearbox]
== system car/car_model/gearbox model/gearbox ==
  note: "feedback" from the propeller shaft
  note: "feedback" to the clutch
  ctrl : Inport
  mech power in [Nm] : Inport  Port=2
  mech fb in [rad/s] : Inport  Port=3
  Bus Creator : BusCreator  Inputs=2
  Bus Creator5 : BusCreator  Inputs=2
  Bus Selector1 : BusSelector  OutputSignals=speed [rad/s],angle [rad]
  Bus Selector2 : BusSelector  OutputSignals=gear ratio,gear inertia
  Bus Selector5 : BusSelector  OutputSignals=torque [Nm],inertia [kg m^2]
  Constant : Constant  Value=mass
  Gain : Gain  Gain=b_t
  Product : Product  Inputs=**  SaturateOnIntegerOverflow=on
  Product1 : Product  Inputs=**  SaturateOnIntegerOverflow=on
  Product2 : Product  SaturateOnIntegerOverflow=on
  Product3 : Product  Inputs=3  SaturateOnIntegerOverflow=on
  Sum : Sum  Inputs=++|
  Sum1 : Sum  Inputs=+-
  Terminator : Terminator
  sensor out : Outport
  mech power out [Nm] : Outport  Port=2
  mech fb out [rad/s] : Outport  Port=3
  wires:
  Bus Creator5/1 -> mech fb out [rad/s]/1
  Product1/1 -> Bus Creator5/2  "angle [rad]"
  Product/1 -> Bus Creator5/1  "speed [rad/s]"
  Bus Selector5/2 -> Product3/3  "<inertia [kg m^2]>"
  Bus Selector5/1 -> Product2/2  "<torque [Nm]>"
  mech power in [Nm]/1 -> Bus Selector5/1
  Bus Selector1/1 -> Product/2, Gain/1  "<speed [rad/s]>"
  Constant/1 -> Terminator/1
  Bus Selector1/2 -> Product1/2  "<angle [rad]>"
  Bus Creator/1 -> mech power out [Nm]/1, sensor out/1
  mech fb in [rad/s]/1 -> Bus Selector1/1
  ctrl/1 -> Bus Selector2/1
  Bus Selector2/1 -> Product2/1, Product3/1, Product3/2, Product/1, Product1/1  "<gear ratio>"
  Product2/1 -> Sum1/1  "i_t T_t"
  Sum1/1 -> Bus Creator/1  "torque [Nm]"
  Gain/1 -> Sum1/2  "b_t omega-t"
  Bus Selector2/2 -> Sum/1  "<gear inertia>"
  Sum/1 -> Bus Creator/2  "inertia [kg m^2]"
  Product3/1 -> Sum/2

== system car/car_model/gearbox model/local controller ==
  cmd in : Inport
  sensor in : Inport  Port=2
  Bus Creator : BusCreator  Inputs=2
  Bus Selector : BusSelector  OutputSignals=gear number
  gear number to inertia table : Lookup  InputValues=gearNumber  Table=gearInertia  LookUpMeth=Interpolation-Use End Values
  gear number to ratio table : Lookup  InputValues=gearNumber  Table=gearRatio  LookUpMeth=Interpolation-Use End Values
  sensor out : Outport
  ctrl : Outport  Port=2
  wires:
  sensor in/1 -> sensor out/1
  cmd in/1 -> Bus Selector/1
  Bus Selector/1 -> gear number to ratio table/1, gear number to inertia table/1  "<gear number>"
  Bus Creator/1 -> ctrl/1
  gear number to ratio table/1 -> Bus Creator/1  "gear ratio"
  gear number to inertia table/1 -> Bus Creator/2  "gear inertia"

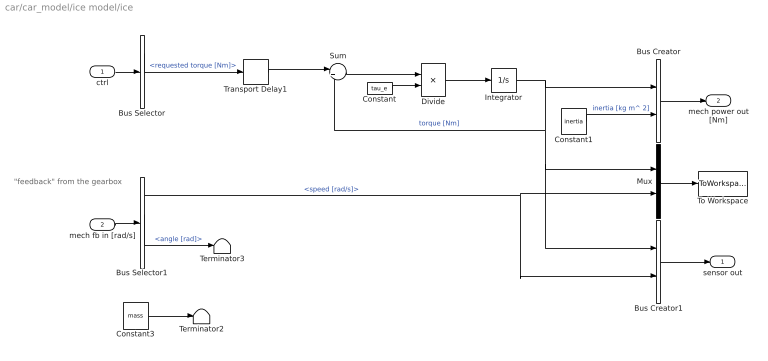
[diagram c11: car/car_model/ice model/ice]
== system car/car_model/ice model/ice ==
  note: "feedback" from the gearbox
  ctrl : Inport
  mech fb in [rad/s] : Inport  Port=2
  Bus Creator : BusCreator  Inputs=2
  Bus Creator1 : BusCreator  Inputs=2
  Bus Selector : BusSelector  OutputSignals=requested torque [Nm]
  Bus Selector1 : BusSelector  OutputSignals=speed [rad/s],angle [rad]
  Constant : Constant  Value=tau_e
  Constant1 : Constant  Value=inertia
  Constant3 : Constant  Value=mass
  Divide : Product  Inputs=*/
  Integrator : Integrator  InitialCondition=init_T
  Mux : Mux  Inputs=2
  Sum : Sum  Inputs=|+-
  Terminator2 : Terminator
  Terminator3 : Terminator
  To Workspace : ToWorkspace  VariableName=iceout  SampleTime=-1
  Transport Delay1 : TransportDelay  DelayTime=tau_d
  sensor out : Outport
  mech power out [Nm] : Outport  Port=2
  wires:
  Constant3/1 -> Terminator2/1
  Bus Creator1/1 -> sensor out/1
  Mux/1 -> To Workspace/1
  Bus Selector1/2 -> Terminator3/1  "<angle [rad]>"
  Bus Creator/1 -> mech power out [Nm]/1
  mech fb in [rad/s]/1 -> Bus Selector1/1
  ctrl/1 -> Bus Selector/1
  Constant/1 -> Divide/2
  Divide/1 -> Integrator/1
  Sum/1 -> Divide/1
  Integrator/1 -> Bus Creator/1, Sum/2, Mux/1, Bus Creator1/1  "torque [Nm]"
  Constant1/1 -> Bus Creator/2  "inertia [kg m^ 2]"
  Bus Selector1/1 -> Mux/2, Bus Creator1/2  "<speed [rad/s]>"
  Bus Selector/1 -> Transport Delay1/1  "<requested torque [Nm]>"
  Transport Delay1/1 -> Sum/1

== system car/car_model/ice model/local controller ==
  cmd in : Inport
  sensor in : Inport  Port=2
  Bus Creator : BusCreator  Inputs=1
  Bus Selector : BusSelector  OutputSignals=torque level
  Bus Selector1 : BusSelector  OutputSignals=speed [rad/s]
  Compare To Constant : simulink/Logic and Bit Operations/Compare To Constant  relop=>=  const=N_max*0.99  OutDataTypeStr=uint8  ZeroCross=off
  Compare To Constant1 : simulink/Logic and Bit Operations/Compare To Constant  relop=<=  const=N_idle*1.15  OutDataTypeStr=uint8  ZeroCross=off
  Idle controller : Subsystem
  Max speed controller : Subsystem
  MinMax : MinMax  Function=max  Inputs=2
  MinMax1 : MinMax  Inputs=2
  Saturation : Saturate  UpperLimit=T_max  LowerLimit=-T_max
  gain : Gain  SaturateOnIntegerOverflow=on
  sensor out : Outport
  ctrl : Outport  Port=2
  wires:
  Max speed controller/1(req_T) -> MinMax1/2
  Compare To Constant/1 -> Max speed controller/Enable
  MinMax/1 -> Bus Creator/1  "requested torque [Nm]"
  [DriverRequstedTorque] -> Idle controller/2(Driver request)
  Compare To Constant1/1 -> Idle controller/Enable
  Idle controller/1(req_T) -> MinMax/2
  Bus Selector1/1 -> Compare To Constant/1, Compare To Constant1/1, Idle controller/1(w_e)  "<speed [rad/s]>"
  gain/1 -> MinMax1/1, [DriverRequstedTorque]
  MinMax1/1 -> MinMax/1
  sensor in/1 -> sensor out/1, Bus Selector1/1
  Bus Creator/1 -> ctrl/1
  Saturation/1 -> gain/1
  Bus Selector/1 -> Saturation/1  "<torque level>"
  cmd in/1 -> Bus Selector/1

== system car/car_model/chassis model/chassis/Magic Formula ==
  note: Note: The SAE definition of the slip ratio kappa is used.
  forward velocity [m/s] : Inport
  wheel speed [rad/s] : Inport  Port=2
  Constant : Constant
  Divide : Product  Inputs=*/
  Gain : Gain  Gain=r_w
  Magic Formula : Fcn  Expr=Dx*sin(Cx*atan(Bx*u-Ex*(Bx*u-atan(Bx*u))))
  Sum3 : Sum  Inputs=-+|
  F_w [N] : Outport
  slip ratio : Outport  Port=2
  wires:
  Gain/1 -> Divide/1
  Sum3/1 -> Magic Formula/1, slip ratio/1  "kappa"
  Constant/1 -> Sum3/1
  Divide/1 -> Sum3/2
  wheel speed [rad/s]/1 -> Gain/1
  Magic Formula/1 -> F_w [N]/1
  forward velocity [m/s]/1 -> Divide/2

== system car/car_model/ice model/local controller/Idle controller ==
  w_e : Inport
  Driver request : Inport  Port=2
  Enable : EnablePort  StatesWhenEnabling=reset  PropagateVarSize=During execution
  Constant : Constant  Value=N_idle
  Gain : Gain  Gain=P
  Gain1 : Gain  Gain=I
  Integrator : Integrator  InitialConditionSource=external
  Sum : Sum  Inputs=+|+
  Sum1 : Sum  Inputs=|-+
  Sum2 : Sum  Inputs=-+|
  req_T : Outport  OutputWhenDisabled=reset  InitialOutput=-T_max
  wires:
  Sum2/1 -> Integrator/2
  Driver request/1 -> Sum2/2
  Constant/1 -> Sum1/2
  Sum1/1 -> Gain1/1, Gain/1
  w_e/1 -> Sum1/1
  Gain/1 -> Sum/1, Sum2/1
  Integrator/1 -> Sum/2
  Gain1/1 -> Integrator/1
  Sum/1 -> req_T/1

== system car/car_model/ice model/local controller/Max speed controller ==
  Enable : EnablePort  StatesWhenEnabling=reset  PropagateVarSize=During execution
  Constant1 : Constant  Value=-T_max
  req_T : Outport  OutputWhenDisabled=reset  InitialOutput=T_max
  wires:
  Constant1/1 -> req_T/1
